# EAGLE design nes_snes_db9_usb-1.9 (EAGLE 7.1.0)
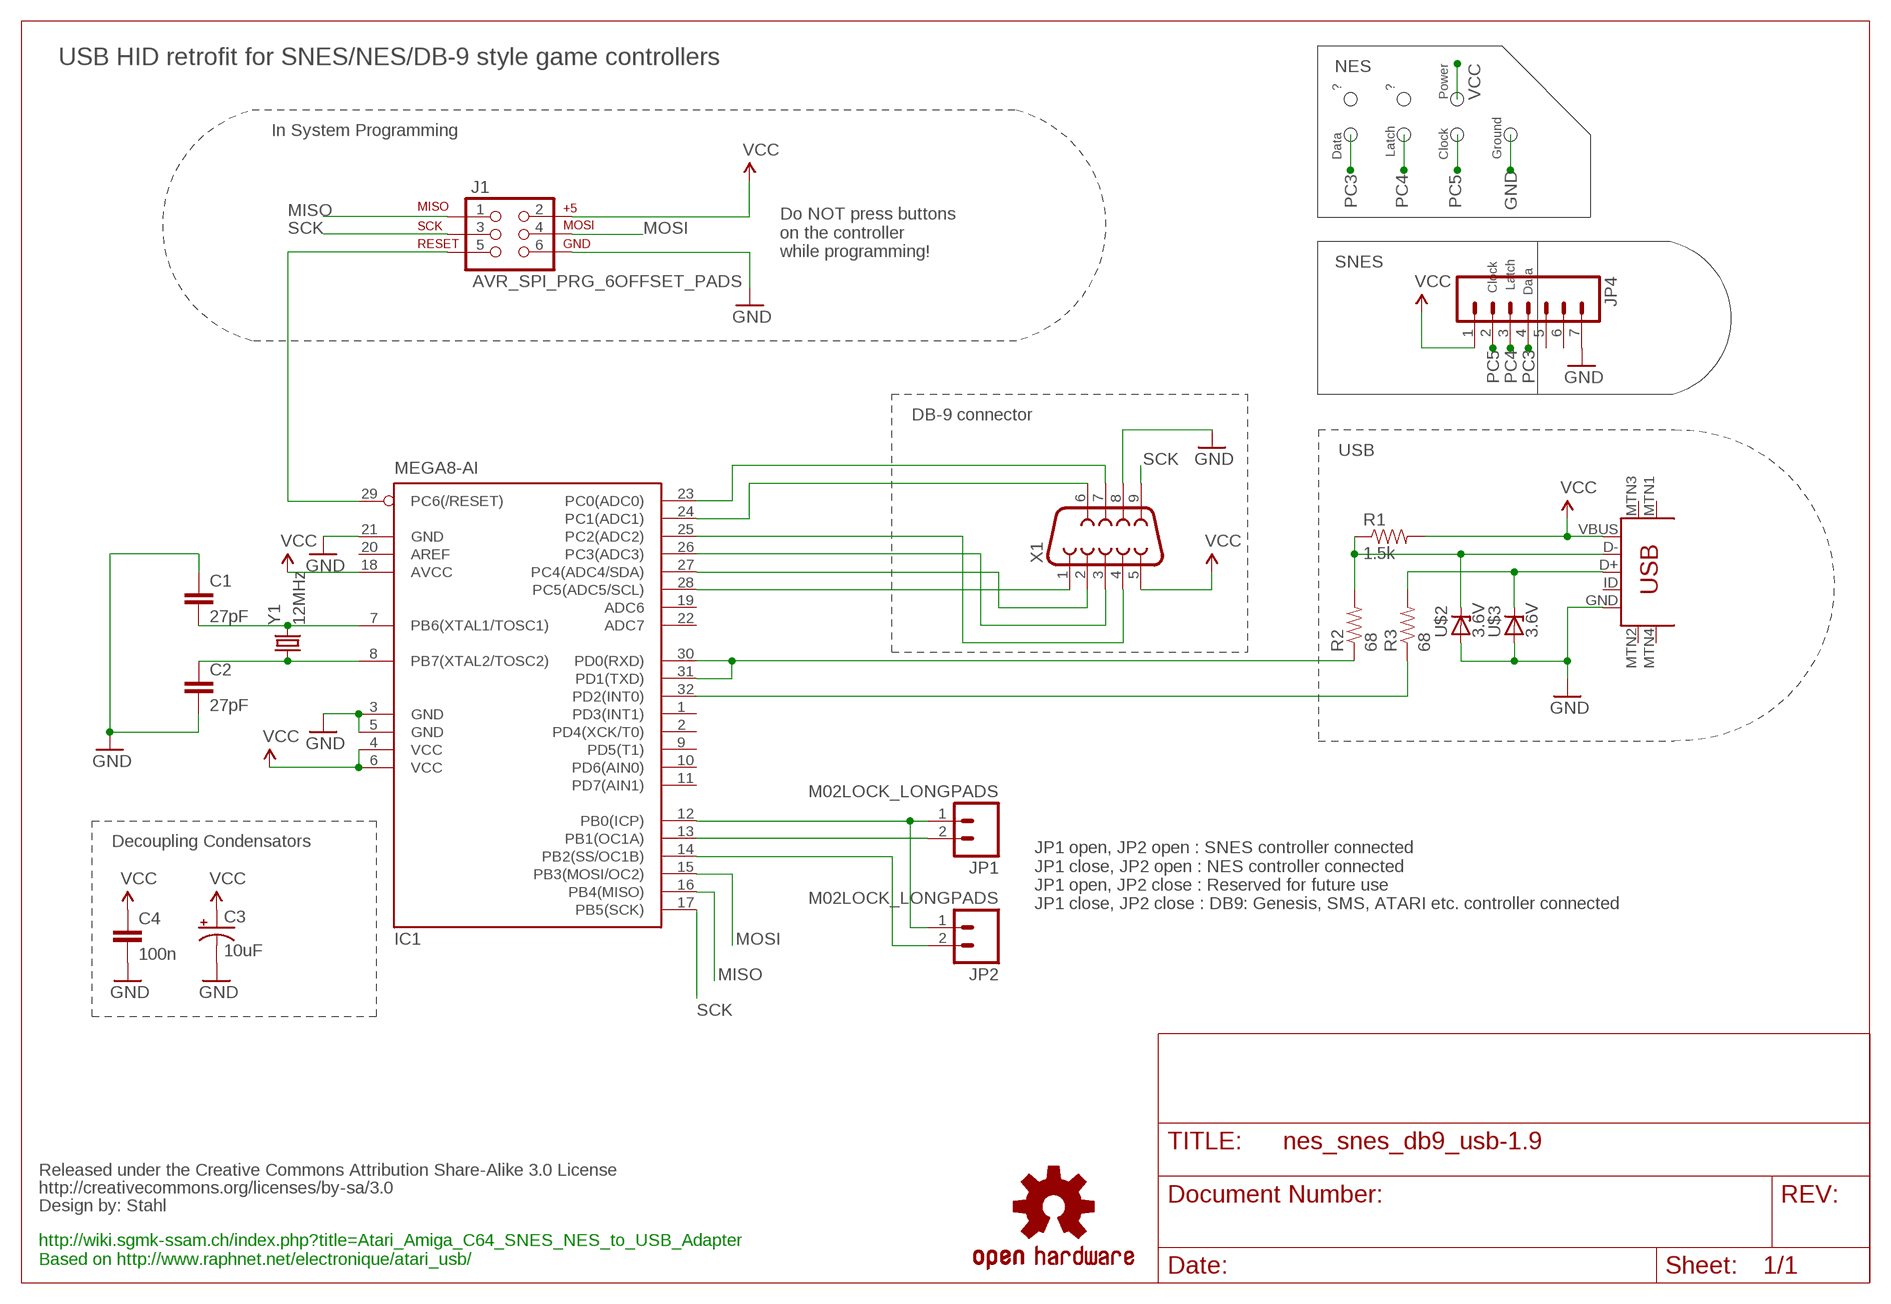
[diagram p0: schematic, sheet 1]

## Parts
C1  27pF  CAP1206  [1206]
C2  27pF  CAP1206  [1206]
C3  10uF  CPOL-USB  [PANASONIC_B]
C4  100n  CAP1206  [1206]
CC_TEXT1  CREATIVE_COMMONS  [CREATIVE_COMMONS]
IC1  MEGA8-AI  [TQFP32-08]
J1  AVR_SPI_PRG_6OFFSET_PADS  [2X3_OFFSET]
JP1  M02LOCK_LONGPADS  [1X02_LOCK_LONGPADS]
JP2  M02LOCK_LONGPADS  [1X02_LOCK_LONGPADS]
JP4  M07  [1X07]
LOGO1  OSHW-LOGOL  [OSHW-LOGO-L]
R1  1.5k  RESISTOR1206  [1206]
R2  68  RESISTOR1206  [1206]
R3  68  RESISTOR1206  [1206]
U$1  USB-MINIB-5PIN  [USB-MINIB]
U$2  3.6V  ZENER-DIODESOD80C  [SOD80C]
U$3  3.6V  ZENER-DIODESOD80C  [SOD80C]
X1  DB9MALE  [DB9_MALE]
Y1  12MHz  CRYSTALSMD  [HC49UP]

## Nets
D+: R3.2 U$1.D+ U$3.C
D-: R1.1 R2.2 U$1.D- U$2.C
GND: C1.1 C2.2 C3.- C4.2 IC1.3(GND) IC1.5(GND) IC1.21(GND) J1.6 JP4.7 U$1.GND U$2.A U$3.A X1.8
MISO: IC1.16(PB4(MISO)) J1.1
MOSI: IC1.15(PB3(MOSI/OC2)) J1.4
N$2: C1.2 IC1.7(PB6(XTAL1/TOSC1)) Y1.2
N$3: C2.1 IC1.8(PB7(XTAL2/TOSC2)) Y1.1
N$6: IC1.12(PB0(ICP)) JP1.1 JP2.1
N$7: IC1.13(PB1(OC1A)) JP1.2
N$8: IC1.14(PB2(SS/OC1B)) JP2.2
N$10: IC1.30(PD0(RXD)) IC1.31(PD1(TXD)) R2.1
N$12: IC1.32(PD2(INT0)) R3.1
PC0: IC1.23(PC0(ADC0)) X1.7
PC1: IC1.24(PC1(ADC1)) X1.6
PC2: IC1.25(PC2(ADC2)) X1.4
PC3: IC1.26(PC3(ADC3)) JP4.4 X1.3
PC4: IC1.27(PC4(ADC4/SDA)) JP4.3 X1.2
PC5: IC1.28(PC5(ADC5/SCL)) JP4.2 X1.1
RESET: IC1.29(PC6(/RESET)) J1.5
SCK: IC1.17(PB5(SCK)) J1.3 X1.9
VCC: C3.+ C4.1 IC1.4(VCC) IC1.6(VCC) IC1.18(AVCC) J1.2 JP4.1 R1.2 U$1.VBUS X1.5
Unconnected: IC1.1(PD3(INT1)) IC1.2(PD4(XCK/T0)) IC1.9(PD5(T1)) IC1.10(PD6(AIN0)) IC1.11(PD7(AIN1)) IC1.19(ADC6) IC1.20(AREF) IC1.22(ADC7) JP4.5 JP4.6 U$1.ID U$1.MTN1(MTN2) U$1.MTN2(MTN3) U$1.MTN3(MTN1) U$1.MTN4

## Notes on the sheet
- USB HID retrofit for SNES/NES/DB-9 style game controllers
- NES
- ? | ?
- Power
- Ground
- Latch | Clock
- Data
- In System Programming
- Do NOT press buttons
  on the controller
  while programming!
- Clock | Latch
- SNES | Data
- DB-9 connector
- USB
- Decoupling Condensators
- JP1 open, JP2 open : SNES controller connected
  JP1 close, JP2 open : NES controller connected
  JP1 open, JP2 close : Reserved for future use
  JP1 close, JP2 close : DB9: Genesis, SMS, ATARI etc. controller connected
- http://wiki.sgmk-ssam.ch/index.php?title=Atari_Amiga_C64_SNES_NES_to_USB_Adapter
  Based on http://www.raphnet.net/electronique/atari_usb/

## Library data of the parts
C1 C2 C4 = SparkFun-Capacitors:CAP: Capacitor
C3 = adafruit:CPOL-US: POLARIZED CAPACITOR, American symbol
CC_TEXT1 = SparkFun-Aesthetics:CREATIVE_COMMONS: Creative Commons License summary
IC1 = atmel:MEGA8: MICROCONTROLLER 8 Kbytes FLASH, 1 kbytes SRAM, 512 bytes EEPROM, USART, 6-channel 10 bit ADC, 2-channel 8 bit ADC Pin compatible with Atmega48, ATMega88, ATMega168 Source: avr.lbr; MPN: ATMEGA8-16AU; OC_FARNELL: 9171371; OC_NEWARK: 73M8863
J1 = SparkFun-Connectors:AVR_SPI_PRG_6: AVR ISP 6 Pin This is the reduced ISP connector for AVR programming. Common on Arduino. This footprint will take up less PCB space and can be used with a 10-pin to 6-pin adapter such as SKU: BOB-08508
JP1 JP2 = SparkFun-Connectors:M02: Standard 2-pin 0.1" header. Use with
JP4 = SparkFun-Connectors:M07: Header 7 Standard 7-pin 0.1" header. Use with straight break away headers (SKU : PRT-00116), right angle break away headers (PRT-00553), swiss pins (PRT-00743), machine pins (PRT-00117), and female headers (PRT-00115). NOTES ON THE VARIANTS LOCK and LOCK_LONGPADS... This footprint was designed to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
LOGO1 = SparkFun-Aesthetics:OSHW-LOGO: Open Source Hardware Logo This logo indicates the piece of hardware it is found on incorporates a OSHW license and/or adheres to the definition of open source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
R1-R3 = SparkFun-Resistors:RESISTOR: Resistor
U$1 = SparkFun-Connectors:USB-MINIB: Mini-USB "B" connector with 5th pin broken out. Created new symbol breaking out 5th "ID" pin in mini/micro USB connector spec. See: http://en.wikipedia.org/wiki/Mini_usb#Cables. Uses same footprint as 4-pin symbol. Also added pins to connect to mounting / shield pads if required (probably not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
U$2 U$3 = diode:ZENER-DIODE: Z-Diode
X1 = SparkFun-Connectors:DB9: DB9 Connector Standard DB9 (D-Sub 9) serial connector. Can be used for CAN bus as well as RS485 and RS232. Footprint production proven. Spark Fun Electronics SKU : PRT-00429
Y1 = SparkFun-FreqCtrl:CRYSTAL: Various standard crystals. Proven footprints. Spark Fun Electronics SKU : COM-00534

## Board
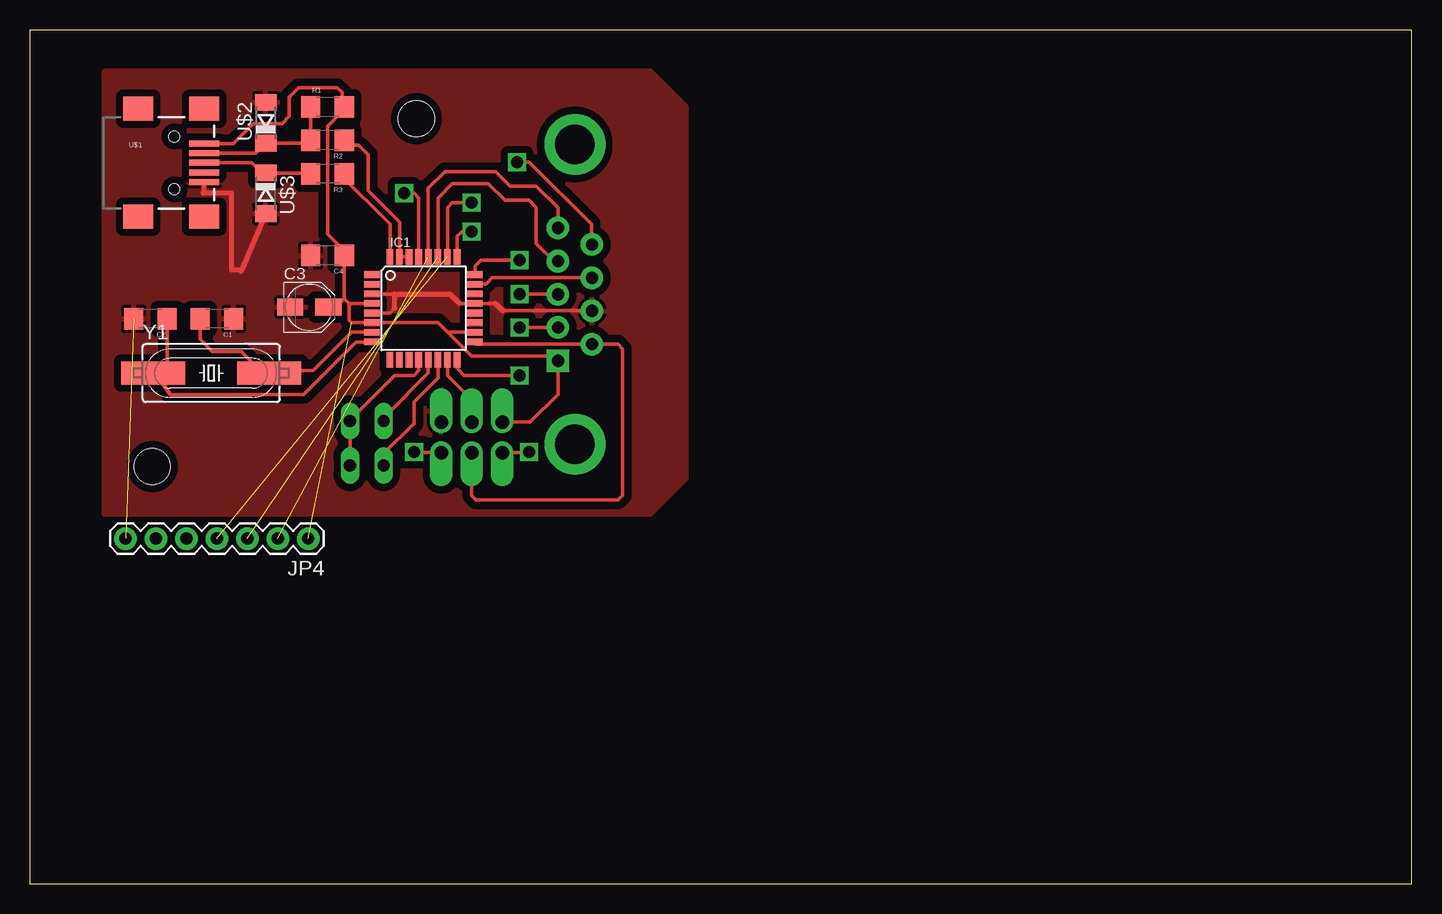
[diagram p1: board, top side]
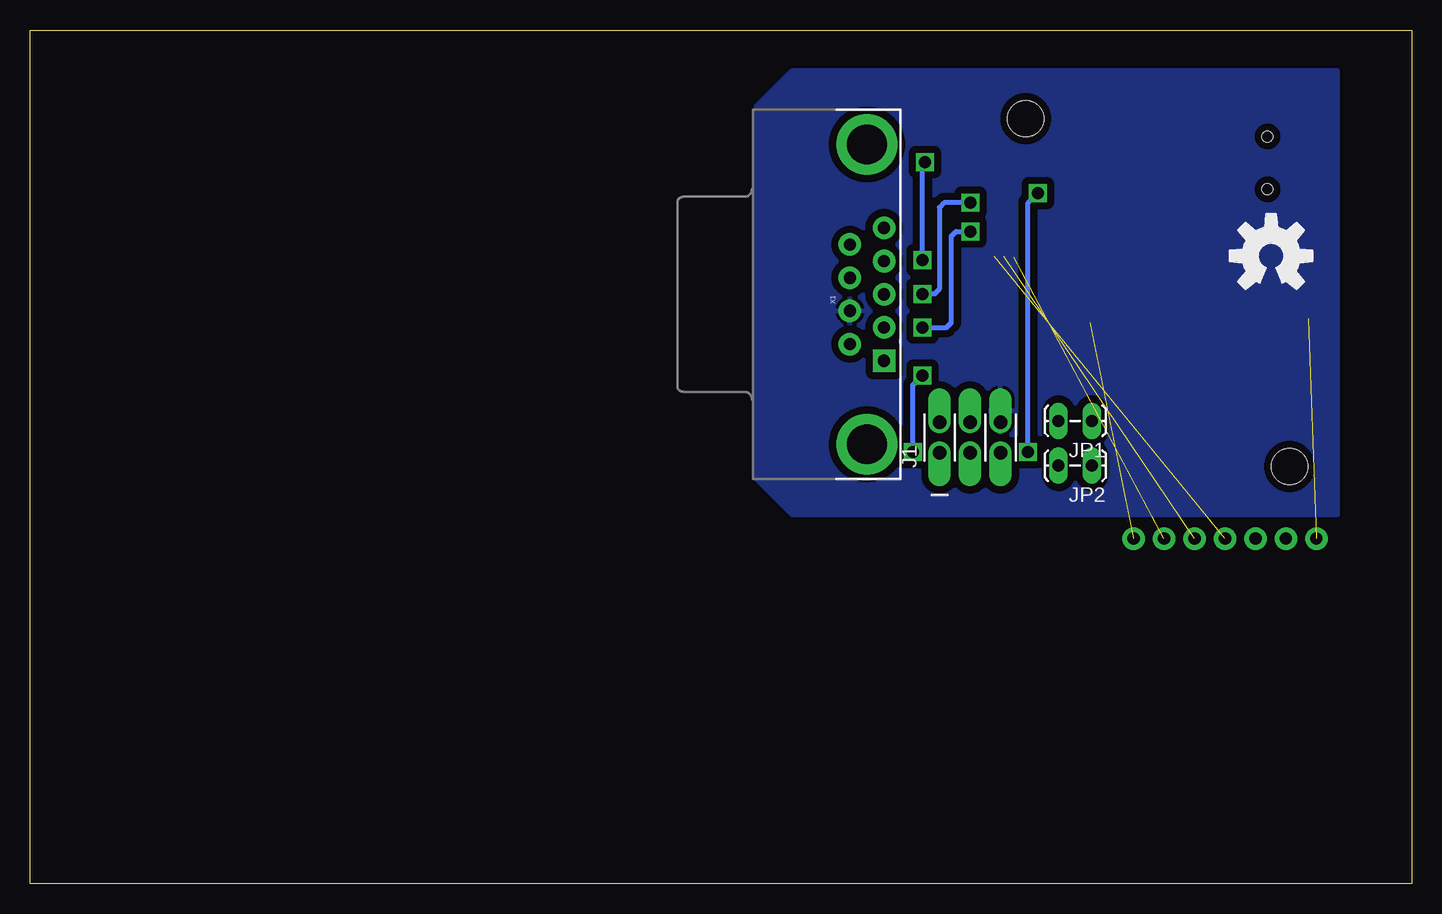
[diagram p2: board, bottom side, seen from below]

Size 115.2 x 71.2 mm. Coordinates in mm from the lower left corner, seen from the top.
Outline: 0,0 115.2,0 115.2,71.2 0,71.2 0,0
Copper layers (1*16): Top 0.035mm / dielectric 1.5mm / Bottom 0.035mm
Design rules "SeeedStudio_2layer_DRU_no_angle_20140221": minimum track width 6mil, minimum drill 12mil, track to track 6mil, track to pad 6mil, pad to pad 6mil, via to via 6mil, smd to smd 0mil, copper to edge 10mil, drill to drill 10mil, minimum pad ring 10mil, minimum via ring 6mil, stop-mask expansion 2mil, vias tented up to drill 100mil, thermal gap 10mil
Holes 3 mm at 32.2,63.8 10.2,34.8

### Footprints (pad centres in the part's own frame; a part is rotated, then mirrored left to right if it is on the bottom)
1206 = smd 1.6 x 1.8: 1 -1.4,0; 2 1.4,0
PANASONIC_B = smd 2.2 x 1.4: + 1.6,0; - -1.6,0
TQFP32-08 = smd 1.27 x 0.559: 1 -4.293,2.8; 2 -4.293,2; 3 -4.293,1.2; 4 -4.293,0.4; 5 -4.293,-0.4; 6 -4.293,-1.2; 7 -4.293,-2; 8 -4.293,-2.8; 17 4.293,-2.8; 18 4.293,-2; 19 4.293,-1.2; 20 4.293,-0.4; 21 4.293,0.4; 22 4.293,1.2; 23 4.293,2; 24 4.293,2.8 | smd 0.559 x 1.27: 9 -2.8,-4.293; 10 -2,-4.293; 11 -1.2,-4.293; 12 -0.4,-4.293; 13 0.4,-4.293; 14 1.2,-4.293; 15 2,-4.293; 16 2.8,-4.293; 25 2.8,4.293; 26 2,4.293; 27 1.2,4.293; 28 0.4,4.293; 29 -0.4,4.293; 30 -1.2,4.293; 31 -2,4.293; 32 -2.8,4.293
2X3_OFFSET = drill 1.118 pad 1.88 offset: 1 -2.54,-1.27; 2 -2.54,1.27; 3 0,-1.27; 4 0,1.27; 5 2.54,-1.27; 6 2.54,1.27
1X02_LOCK_LONGPADS = drill 1.016 long: 1 -0.127,0; 2 2.667,0
1X07 = drill 1.016 pad 1.88: 1 0,0; 2 2.54,0; 3 5.08,0; 4 7.62,0; 5 10.16,0; 6 12.7,0; 7 15.24,0
USB-MINIB = smd 2.5 x 0.5: D+ 2.5,0; D- 2.5,0.8; GND 2.5,-1.6; ID 2.5,-0.8; VBUS 2.5,1.6 | smd 2.5 x 2: MTN1 -3,4.5; MTN2 2.5,4.5; MTN3 -3,-4.5; MTN4 2.5,-4.5 | hole 0.9: 0,2.2; 0,-2.2
SOD80C = smd 1.4 x 1.8: A 1.7,0; C -1.7,0
DB9_MALE = drill 1.016 pad 1.88: 1 5.54,-1.42; 2 2.77,-1.42; 3 0,-1.42; 4 -2.77,-1.42; 6 4.15,1.42; 7 1.38,1.42; 8 -1.38,1.42; 9 -4.15,1.42 | drill 1.016 pad 1.88 square: 5 -5.54,-1.42 | drill 3.302 pad 5.08: G1 -12.5,0; G2 12.5,0
HC49UP = smd 5.334 x 1.93: 1 -4.826,0; 2 4.826,0

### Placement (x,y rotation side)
C1  15.59,47.12 180 top
C2  10.04,47.12 180 top
C3  23.29,48.09 0 top
C4  24.8,52.4 180 top
CC_TEXT1  23.98,2.5 0 top
IC1  32.8,48 0 top
J1  36.83,37.23 0 bottom
JP1  26.8,38.6 180 bottom
JP2  26.8,34.88 180 bottom
JP4  23.2,28.8 180 top
LOGO1  11.74,52.36 0 bottom
R1  24.8,64.8 0 top
R2  24.8,62 180 top
R3  24.8,59.2 180 top
U$1  12.04,60.12 0 top
U$2  19.66,63.46 90 top
U$3  19.66,57.58 270 top
X1  45.43,49.16 90 bottom
Y1  15.11,42.6 0 top

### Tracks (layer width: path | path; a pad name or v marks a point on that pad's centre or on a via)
D+
  Top 0.305: U$1.D+ 18.48,60.12 19.6,59 | U$3.C 23.12,59.28
  Top 0.406: 19.6,59 U$3.C | 23.12,59.28 23.2,59.2 R3.2
D-
  Top 0.305: U$1.D- 18.82,60.92 U$2.C 23.14,61.76 | R2.2 R1.1
  Top 0.406: 23.14,61.76 R2.2
GND  (1 unrouted)
  Top 0.305: IC1.3 30.38,49.2 | 35.8,48.4 IC1.21 38.8,48.4 | IC1.5 30,47.6 30.4,48 | 39.4,47.8 46.83,47.8
  Top 0.406: 30.38,49.2 35,49.2 35.8,48.4 | 30.38,49.2 30.38,48.82 | 30.4,48 30.4,49.18 30.38,49.2 | U$3.A 17.6,51.08 17.6,51.2 16.8,51.2 16.8,57.6 14.54,57.6 | 14.4,57.6 14.54,57.6 | 14.54,57.6 U$1.GND | 38.8,48.4 39.4,47.8 | 46.83,47.8 X1.8
  pour Top (isolate 0.61): 6.2,67.8 51.7,67.8 54.7,64.8 54.7,33.8 51.7,30.8 6.2,30.8
  pour Bottom (isolate 0.61): 6.2,67.8 51.7,67.8 54.7,64.8 54.7,33.8 51.7,30.8 6.2,30.8
MISO  (via drill 1)
  Top 0.305: J1.1 41.56,35.96 | v40.8,42.4 36.2,42.4 35.6,43 IC1.16
  Top 0.406: 41.56,35.96 v41.6,36
  Bottom 0.406: v41.6,36 41.6,41.6 v40.8,42.4
MOSI
  Top 0.305: J1.4 36.83,40.37 34.8,42.4 IC1.15
N$2
  Top 0.305: IC1.7 26.8,46 23.6,42.8 20.14,42.8 | C1.2 14.19,45.41 15.2,44.4 17.6,44.4 18.4,43.6 18.4,42.8
  Top 0.406: 20.14,42.8 Y1.2 19.34,42 19.2,42 18.4,42.8
N$3
  Top 0.305: IC1.8 27.2,45.2 22.8,40.8 11.68,40.8 10.88,42 | C2.1 11.44,42.24
  Top 0.406: 12.24,42.24 12,42 11.2,42 | 11.2,42 10.88,42 Y1.1 | 11.44,42.24 11.2,42
N$6
  Top 0.305: JP2.1 JP1.1 26.67,38.67 30.4,42.4 32,42.4 32.4,42.8 IC1.12
N$7
  Top 0.305: IC1.13 33.2,42.6 29.8,39.2 29.5,38.93 JP1.2
N$8
  Top 0.305: JP2.2 29.47,35.87 32,38.4 32,40.2 34,42.2 IC1.14
N$10
  Top 0.305: IC1.30 IC1.31 30.8,55.2 28.2,57.8 28.2,60.8 27.4,61.6 26.6,61.6
  Top 0.406: 26.6,61.6 R2.1
N$12
  Top 0.305: IC1.32 30,55 25.8,59.2
  Top 0.406: 26.16,59.4 R3.1 25.8,59.2
PC0
  Top 0.305: X1.7 38.54,50.54 38,50 IC1.23
PC1  (via drill 1)
  Top 0.305: IC1.24 37.09,51.49 37.6,52 v40.8,52 | v40.6,60.2 41.6,60.2 46.8,55 46.8,53.36
  Top 0.406: 46.8,53.36 X1.6
  Bottom 0.406: v40.8,52 40.8,59.8 v40.6,60.2
PC2  (via drill 1)
  Top 0.305: X1.4 41.61,46.39 v40.8,46.4 | v36.8,54.4 36,54.4 35.6,54 IC1.25
  Bottom 0.406: v40.8,46.4 38.8,46.4 38.4,46.8 38.4,54 38,54.4 v36.8,54.4
PC3  (via drill 1)  (1 unrouted)
  Top 0.305: IC1.26 34.8,56.4 35.2,56.8 v36.8,56.8 | v40.8,49.2 43.97,49.2
  Top 0.406: 43.97,49.2 X1.3
  Bottom 0.406: v36.8,56.8 39,56.8 39.4,56.4 39.4,49.6 39.8,49.2 v40.8,49.2
PC4  (1 unrouted)
  Top 0.305: IC1.27 34,57.2 35.2,58.4 38.2,58.4 39.6,57 41.6,57 42.2,56.4 42.2,53.4 43.8,51.8 43.94,52 X1.2
PC5  (1 unrouted)
  Top 0.305: X1.1 44.01,56.39 42.2,58.2 40,58.2 38.8,59.4 34.6,59.4 33.2,58 IC1.28
  Top 0.406: 33.2,52.25 IC1.28
RESET  (via drill 1)
  Top 0.305: J1.5 32.04,35.96 | v31.2,57.6 32,57.6 32.4,57.2 IC1.29
  Top 0.406: 32.04,35.96 v32,36
  Bottom 0.406: v32,36 32,56.8 v31.2,57.6
SCK
  Top 0.305: X1.9 37.1,45.01 IC1.17 | J1.3 36.83,32.37 37.2,32 49,32 49.4,32.4 49.4,44.6 49,45 X1.9
  Top 0.406: X1.9
VCC  (1 unrouted)
  Top 0.305: J1.2 41.7,38.5 44,40.8 X1.5 | 34.8,46 34,46.8 IC1.6 26.8,46.8 26.6,47 26.6,48.4 | 34.8,46 36.8,44 43.63,44 X1.5 | IC1.18 34.8,46 | U$1.VBUS 16.92,61.72 18.6,63.4 21,63.4 21.6,64 21.6,65.6 22.4,66.4 25.6,66.4 26,66 26,64.87 | 26.2,64.6 24.8,63.2 24.8,54.2 26.2,52.8 | IC1.4 26.6,48.4 | 26.6,48.4 26.2,48.8 | 26.2,48.8 C4.1 | 26.2,48.8 25.8,48.4 24.2,48.4
  Top 0.406: X1.5 | 26,64.87 R1.2 26.2,64.6 | 26.2,52.8 26.6,51.8 25.8,52.8 C4.1 | 24.2,48.4 C3.+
